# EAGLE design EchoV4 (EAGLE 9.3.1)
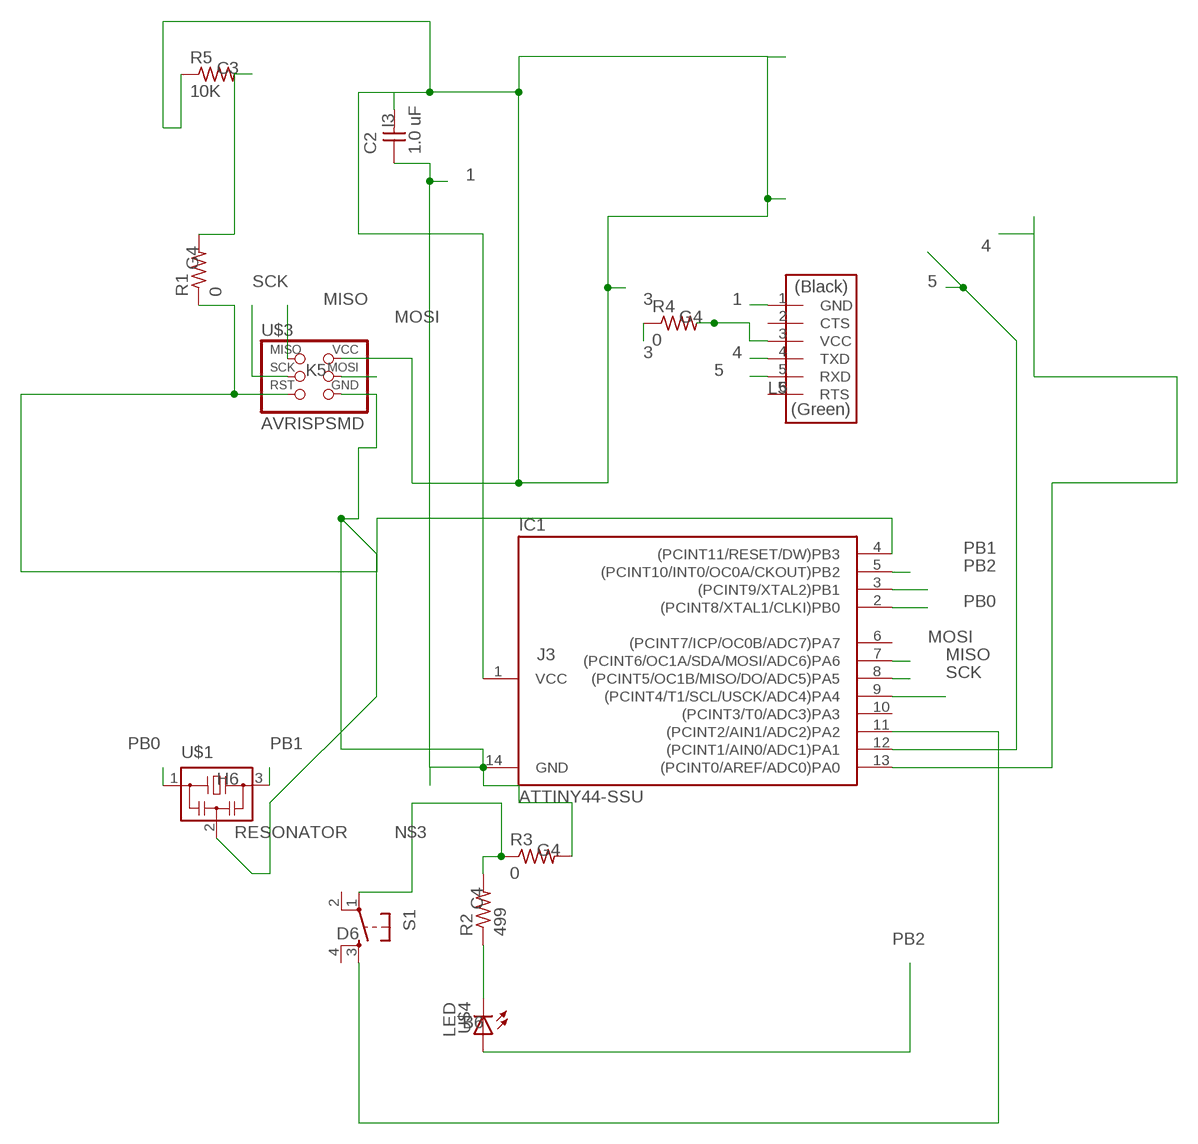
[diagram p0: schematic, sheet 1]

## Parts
C2  1.0 uF  CAP-UNPOLARIZEDFAB  [C1206FAB]
IC1  ATTINY44-SSU  [SOIC14]
R1  0  RES-US1206FAB  [R1206FAB]
R2  499  RES-US1206  [R1206]
R3  0  RES-US1206  [R1206]
R4  0  RES-US1206  [R1206]
R5  10K  RES-US1206  [R1206]
S1  6MM_SWITCH6MM_SWITCH  [6MM_SWITCH]
U$1  RESONATOR  [EFOBM]
U$2  FTDI-SMD-HEADER  [1X06SMD]
U$3  AVRISPSMD  [2X03SMD]
U$4  LED  [LED1206]

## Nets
1: C2.1 IC1.14(GND) R3.2 U$1.2 U$2.1(GND) U$3.6(GND)
3: C2.2 IC1.1(VCC) R4.1 R4.2 R5.1 U$2.3(VCC) U$3.2(VCC)
4: IC1.13((PCINT0/AREF/ADC0)PA0) U$2.4(TXD)
5: IC1.12((PCINT1/AIN0/ADC1)PA1) U$2.5(RXD)
MISO: IC1.8((PCINT5/OC1B/MISO/DO/ADC5)PA5) U$3.1(MISO)
MOSI: IC1.7((PCINT6/OC1A/SDA/MOSI/ADC6)PA6) U$3.4(MOSI)
N$1: R2.1 U$4.2(C)
N$2: IC1.4((PCINT11/RESET/DW)PB3) R1.1 U$3.5(RST)
N$3: R2.2 R3.1 S1.1(P)
N$4: R1.2 R5.2
N$5: IC1.11((PCINT2/AIN1/ADC2)PA2) S1.3(S)
PB0: IC1.2((PCINT8/XTAL1/CLKI)PB0) U$1.1
PB1: IC1.3((PCINT9/XTAL2)PB1) U$1.3
PB2: IC1.5((PCINT10/INT0/OC0A/CKOUT)PB2) U$4.1(A)
SCK: IC1.9((PCINT4/T1/SCL/USCK/ADC4)PA4) U$3.3(SCK)
Unconnected: IC1.6((PCINT7/ICP/OC0B/ADC7)PA7) IC1.10((PCINT3/T0/ADC3)PA3) S1.2(P1) S1.4(S1) U$2.2(CTS) U$2.6(RTS)

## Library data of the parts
C2 = eagle_fab:CAP-UNPOLARIZED; LOCATION: I3
IC1 = eagle_fab:ATTINY44; LOCATION: J3
R1 R3 R4 = eagle_fab:RES-US: Resistor (US Symbol); LOCATION: G4
R2 = eagle_fab:RES-US: Resistor (US Symbol); LOCATION: C4
R5 = eagle_fab:RES-US: Resistor (US Symbol); LOCATION: C3
S1 = eagle_fab:6MM_SWITCH: OMRON SWITCH; LOCATION: D6
U$1 = eagle_fab:RESONATOR; LOCATION: H6
U$2 = eagle_fab:FTDI-SMD-HEADER; LOCATION: L5
U$3 = eagle_fab:AVRISP; LOCATION: K5
U$4 = eagle_fab:LED: LED; LOCATION: B6

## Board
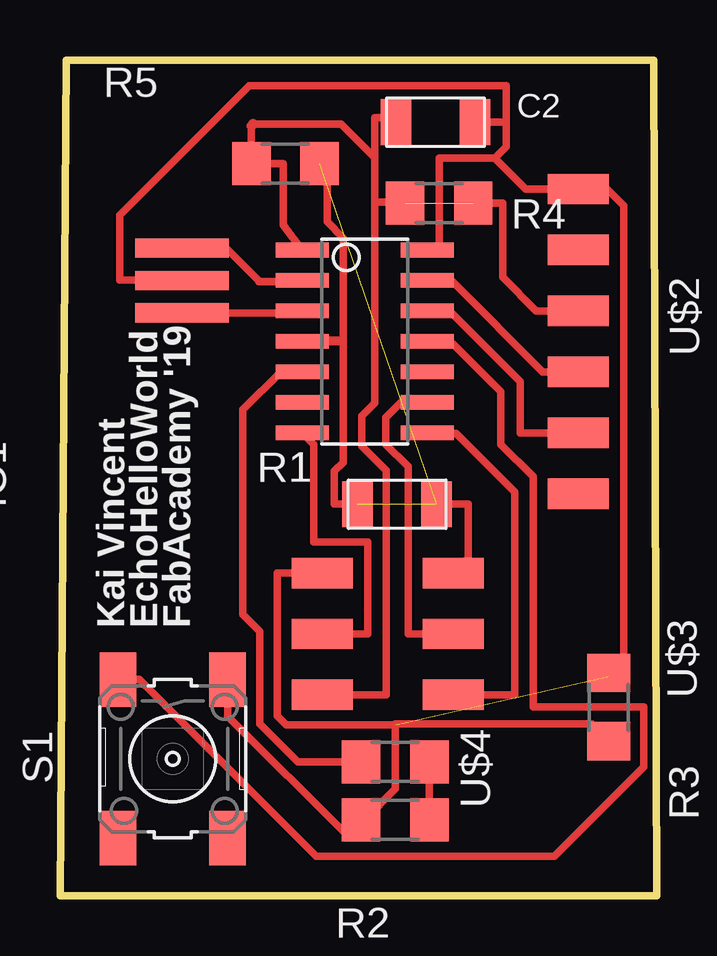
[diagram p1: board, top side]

Size 24.87 x 34.85 mm. Coordinates in mm from the lower left corner, seen from the top.
Outline: 0,0 24.87,0 24.75,34.85 0.25,34.85 0,0
Copper layers (1*16): Top 0.035mm / dielectric 1.5mm / Bottom 0.035mm
Design rules "OthermillDRC_1_64_v2": minimum track width 16mil, minimum drill 31mil, track to track 0.39878125mm, track to pad 0.39878125mm, pad to pad 0.39878125mm, via to via 0.39878125mm, smd to smd 0mil, copper to edge 0mil, drill to drill 1mil, minimum pad ring 0mil, minimum via ring 15mil, stop-mask expansion 1mil, vias tented up to drill 30mil, thermal gap 10mil

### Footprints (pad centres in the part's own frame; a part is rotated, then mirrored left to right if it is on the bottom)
C1206FAB = smd 1.27 x 1.905: 1 -1.651,0; 2 1.651,0
SOIC14 = smd 0.61 x 2.21: 1 -3.81,-2.603; 2 -2.54,-2.603; 3 -1.27,-2.603; 4 0,-2.603; 5 1.27,-2.603; 6 2.54,-2.603; 7 3.81,-2.603; 8 3.81,2.603; 9 2.54,2.603; 10 1.27,2.603; 11 0,2.603; 12 -1.27,2.603; 13 -2.54,2.603; 14 -3.81,2.603
R1206FAB = smd 1.27 x 1.905: 1 -1.651,0; 2 1.651,0
R1206 = smd 1.6 x 1.803: 1 -1.422,0; 2 1.422,0
6MM_SWITCH = smd 2.286 x 1.524: 1 -3.302,2.286; 2 3.302,2.286; 3 -3.302,-2.286; 4 3.302,-2.286
EFOBM = smd 0.8 x 3.9: 1 -1.35,0; 2 0,0; 3 1.35,0
1X06SMD = smd 2.54 x 1.27: 1 0,6.35; 2 0,3.81; 3 0,1.27; 4 0,-1.27; 5 0,-3.81; 6 0,-6.35
2X03SMD = smd 2.54 x 1.27: 1 -2.54,2.54; 2 2.92,2.54; 3 -2.54,0; 4 2.92,0; 5 -2.54,-2.54; 6 2.92,-2.54
LED1206 = smd 1.6 x 1.803: 1 -1.422,0; 2 1.422,0

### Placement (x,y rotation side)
C2  15.65,32.26 180 top
IC1  12.7,23.11 270 top
R1  14.05,16.33 0 top
R2  13.97,3.18 180 top
R3  22.86,7.87 90 top
R4  15.8,28.88 0 top
R5  9.4,30.53 0 top
S1  4.7,5.71 270 top
U$1  5.08,25.65 270 top
U$2  21.59,23.11 0 top
U$3  13.84,10.92 180 top
U$4  13.97,5.59 0 top

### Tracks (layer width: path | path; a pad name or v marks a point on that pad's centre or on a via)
1  (1 unrouted)
  Top 0.305: 22.86,9.14 R3.2 | 18.11,30.76 15.79,30.76 15.79,26.94 15.77,26.92 IC1.14 | 18.11,30.76 19.41,29.46 U$2.1 22.81,29.46 23.5,28.78 23.5,9.93 R3.2 | R3.2 | 5.05,25.68 2.49,25.68 2.49,28.38 7.89,33.78 18.59,33.78 18.59,32.26 | U$3.6 9.05,13.46 9.05,7.51 9.42,7.14 13.97,7.14 | 18.59,32.26 C2.1 | 18.11,30.76 18.59,31.24 18.59,32.26
  Top 0.406: 5.05,25.68 U$1.2
3  (1 unrouted)
  Top 0.305: 13.11,30.79 11.71,32.18 8.05,32.18 | IC1.1 9.31,27.97 9.31,30.52 7.99,30.52 | 13.11,30.79 13.11,32.44 13.82,32.44 | 13.11,30.79 13.11,28.93 | 13.11,28.93 13.11,20.55 12.56,20.01 12.56,18.76 13.59,17.73 13.59,8.38 U$3.2 | 20.85,24.38 U$2.3 19.85,24.38 18.44,25.79 18.44,28.88 R4.2 | 14.33,28.93 13.11,28.93 | 7.98,32.11 R5.1
  Top 0.406: R4.1 14.33,28.93 | 13.82,32.44 C2.2 | 8.05,32.18 7.98,32.11 | 7.99,30.52 R5.1
4
  Top 0.305: IC1.13 15.39,25.6 16.36,25.6 20.12,21.84 U$2.4
5
  Top 0.305: IC1.12 16.23,24.38 19.18,21.44 19.18,19.3 U$2.5
MISO
  Top 0.305: U$3.1 18.96,8.38 18.96,16.83 16.51,19.28 15.33,19.28
  Top 0.406: IC1.8 15.33,19.28
MOSI
  Top 0.305: U$3.4 12.82,10.92 12.82,14.76 10.58,14.76 10.58,18.82 IC1.7
N$1
  Top 0.305: R2.1 U$4.2
N$2  (1 unrouted)
  Top 0.305: 11.12,30.63 11.12,28.12 11.81,27.43 11.81,23.16 10.21,23.16 IC1.4 11.8,23.11 11.8,18.07 11.43,17.7 11.43,16.33 R1.1 | U$3.5 17.02,14.1 17.02,16.33 15.65,16.33
N$3
  Top 0.305: 12,2.48 6.99,7.49 S1.1 | R3.1 22.15,7.16 13.97,7.16 13.97,4.47 13.95,4.45 13.95,4.44 12.69,3.18
  Top 0.406: 12.69,3.18 R2.2 12.55,3.02 12,2.48
N$4  (1 unrouted)
N$5
  Top 0.305: IC1.11 15.39,23.01 16.38,23.01 18.36,21.03 18.36,18.82 19.71,17.48 19.71,7.87 24.33,7.87 24.33,5.38 20.6,1.65 10.67,1.65 3.3,9.02 S1.3
PB0
  Top 0.305: IC1.2 10.06,25.6 8.28,25.6 8.28,25.65 6.93,27 U$1.1
PB1
  Top 0.305: U$1.3 10.02,24.3
  Top 0.406: 10.02,24.3 IC1.3
PB2
  Top 0.305: IC1.5 9.2,21.84 7.62,20.27 7.62,11.73 8.33,11.02 8.33,7.16 9.91,5.59 U$4.1
SCK
  Top 0.305: U$3.3 14.5,10.92 14.5,17.89 13.57,18.83 13.57,19.95 14.2,20.57 IC1.9

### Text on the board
tPlace: Kai Vincent / EchoHelloWorld / FabAcademy '19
